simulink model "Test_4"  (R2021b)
settings: Solver=FixedStepAuto  StartTime=0.0  StopTime=1200
undefined symbols (not defined in the file): Ion, Lithium, Pe
libraries: fl_lib x31, nesl_utility x24, sdl_lib x11, simulink x5, simulink_extras x2, spsBatteryLib x1, spsCurrentVoltageSimscapeInterfaceLib x1, slpidlib x1, spspowerguiLib x1
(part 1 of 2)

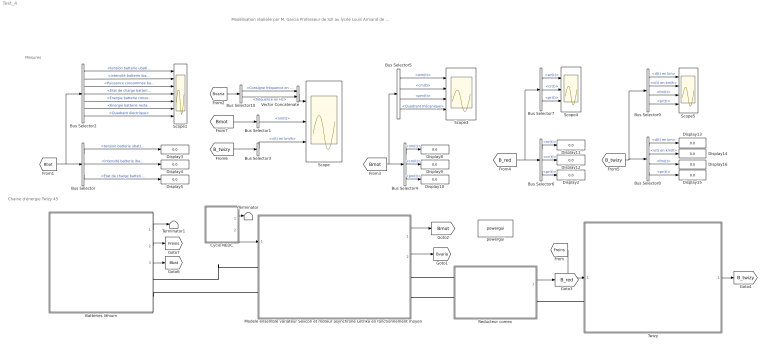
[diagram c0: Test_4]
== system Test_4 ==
  note: Mesures
  note: Chaine d'énergie Twizy 45
  note: Modélisation réalisée par M. Garcia Professeur de S2I au lycée Louis Armand de Nogent sur Marne
  Batteries lithium : Subsystem  mask{Ubat_n=54, Qbat_n=105, Soc_init=100, Soc_min=3}
      mask prompts: Ubat_n "Tension nominale batterie en V"; Qbat_n "Capacité nominale en A.h"; Soc_init "Etat de charge initial"; Soc_min "Seuil minimum en %"
  Bus Selector : BusSelector  OutputSignals=tension batterie ubat(t),intensité batterie ibat(t),Etat de charge batterie soc(t) en %
  Bus Selector1 : BusSelector  OutputSignals=nm(t)
  Bus Selector10 : BusSelector  OutputSignals=Consigne fréquence en Hz,fréquence en Hz
  Bus Selector2 : BusSelector  OutputSignals=tension batterie ubat(t),intensité batterie ibat(t),Puissance consommée batterie pbat(t) en W,Etat de charge batterie soc(t) en %,Energie batterie consommée wbat_cons(t) en Wh,Energie batterie restante wbat_rest(t) en Wh,Quadrant électrique
  Bus Selector3 : BusSelector  OutputSignals=v(t) en km/h
  Bus Selector4 : BusSelector  OutputSignals=nm(t),cm(t),pm(t)
  Bus Selector5 : BusSelector  OutputSignals=wm(t),cm(t),pm(t),Quadrant mécanique
  Bus Selector6 : BusSelector  OutputSignals=nr(t),cr(t),pr(t)
  Bus Selector7 : BusSelector  OutputSignals=wr(t),cr(t),pr(t)
  Bus Selector8 : BusSelector  OutputSignals=d(t) en km,v(t) en km/h,fm(t),pr(t)
  Bus Selector9 : BusSelector  OutputSignals=d(t) en km,v(t) en km/h,fm(t),pr(t)
  Cycle NEDC : Stateflow chart  TreatAsAtomicUnit=on
  Display{2..5,8..16} (13 alike) : Display
  Modele ensemble variateur Sevcon et moteur asynchrone Letrika en fonctionnement moyen : Subsystem  mask{Vbn=52, Tn=33, Nn=2050, fn=68.33, In=120, rend_mot=85, Jm=0.006, f_max_av=190, f_max_ar=54.8, rend_var=92, kp_n=1, ki_n=0.01, pas=0.5}
      mask prompts: Vbn "Tension bobinage nominale moteur en V"; Tn "Couple nominal en N.m"; Nn "Vitesse nominale moteur en tr/min"; fn "fréquence nominale moteur en Hz"; In "Intensité nominale moteur en A"; rend_mot "Rendement moteur en %"; Jm "Moment d'inertie moteur en kg.m²"; f_max_av "Fréquence maximale autorisée en marche avant en hz"; f_max_ar "Fréquence maximale autorisée en marche arrière en hz"; rend_var "Rendement variateur en %"; kp_n "Gain correcteur proportionnel"; ki_n "Gain correcteur intégral"; pas "Réglage pas solveur simscape"
  Reducteur comex : Subsystem  mask{ratio=(68*57)/(17*17), rend_red=96}
      mask prompts: ratio "Rapport de réduction"; rend_red "Rendement moyen transmission en %"
  Scope : Scope  NumInputPorts=3
  Scope1 : Scope  NumInputPorts=7
  Scope3 : Scope  NumInputPorts=4
  Scope4 : Scope  NumInputPorts=3
  Scope5 : Scope  NumInputPorts=4
  Terminator : Terminator
  Terminator1 : Terminator
  Twizy : Subsystem  mask{Vent_de_face=0, Pente=0, n=2, a=746, b=942, h=900, S=1.33, Cx=0.64, M_twizy=375, M_cond=80, M_pass=0, M_Batt=71, t_jantes_av=13, l_pneu_av=125, h_broul_av=80, Prav=2.5, t_jantes_ar=13, l_pneu_ar=145, h_broul_ar=80, Prar=2.5}
      mask prompts: Vent_de_face "Vent de face en km/h"; Pente "Pente de la route en %"; n "Nombre de roue par axe"; a "Distance estimée entre centre de gravitée et l'axe de la roue avant en mm"; b "Distance estimée entre centre de gravité e  et l'axe de la roue arrière en mm"; h "Hauteur estimée du centre de gravité en mm"; S "Surface frontale en m²"; Cx "Coefficient de trainée"; M_twizy "Masse twizy à vide en kg"; M_cond "Masse conducteur en kg"; M_pass "Masse passagers en kg"; M_Batt "Masse batteries en kg"; t_jantes_av "Taille jante en pouces"; l_pneu_av "Largeur en mm"; h_broul_av "Hauteur bande de roulement en %"; Prav "Pression pneus avant en bar"; t_jantes_ar "Taille jante en pouces"; l_pneu_ar "Largeur en mm"; h_broul_ar "Hauteur bande de roulement en %"; Prar "Pression pneus arrière en bar"
  Vector Concatenate : Concatenate
  powergui : spspowerguiLib/powergui  Priority=1  SimulationMode=Discrete  SampleTime=1  frequency=60  Iterations=50  frequencyindice=0  Pbase=100e6  ErrMax=1e-4  UnitsV=kV  UnitsW=MW  buscounter=0  FunctionMessages=off  echomessages=off  EnableUseOfTLC=off  CurrentSourceSwitches=off  DisableSnubberDevices=off  DisableRonSwitches=off  DisableVfSwitches=off  DisplayEquations=off  AutomaticDiscreteSolvers=off  SolverType=Tustin/Backward Euler (TBE)  Interpol=off  ExternalGateDelay=off  methode=off  Ts=100  x0status=blocks  SPID=on  SwTol=0  HookPort=off  NonlinearTolerance=1e-4  nMaxIteration=100  ContinueOnMaxIteration=off  RestoreLinks=warning  ResistiveCurrentMeasurement=off  Frange=[0:2:500]  Ylog=off  Xlog=on  ShowGrid=off  save=off  variable=ZData  structure=0  ZoomFFT=off  StartTime=0.0  cycles=1  DisplayStyle=1  fundamental=60  FreqAxis=off  MaxFrequency=1000  frequencyindicesteady=1  RmsSteady=1  display=off
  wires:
  Reducteur comex/1(Bus) -> [B_red]
  Twizy/1(Bus) -> [B_twizy]
  Modele ensemble variateur Sevcon et moteur asynchrone Letrika en fonctionnement moyen/1(Bus) -> [Bmot]
  Bus Selector/2 -> Display4/1  "<intensité batterie ibat(t)>"
  [Bbat] -> Bus Selector2/1, Bus Selector/1
  Bus Selector9/2 -> Scope5/2  "<v(t) en km/h>"
  Bus Selector9/4 -> Scope5/4  "<pr(t)>"
  Bus Selector8/2 -> Display14/1  "<v(t) en km/h>"
  Bus Selector6/2 -> Display12/1  "<cr(t)>"
  Bus Selector8/3 -> Display16/1  "<fm(t)>"
  Bus Selector7/1 -> Scope4/1  "<wr(t)>"
  Bus Selector8/1 -> Display13/1  "<d(t) en km>"
  Bus Selector4/3 -> Display10/1  "<pm(t)>"
  Bus Selector6/1 -> Display11/1  "<nr(t)>"
  Bus Selector5/3 -> Scope3/3  "<pm(t)>"
  Bus Selector5/2 -> Scope3/2  "<cm(t)>"
  Bus Selector6/3 -> Display2/1  "<pr(t)>"
  Bus Selector5/1 -> Scope3/1  "<wm(t)>"
  Bus Selector4/1 -> Display8/1  "<nm(t)>"
  [B_twizy] -> Bus Selector9/1, Bus Selector8/1
  Bus Selector2/1 -> Scope1/1  "<tension batterie ubat(t)>"
  [Bmot] -> Bus Selector4/1, Bus Selector5/1
  Bus Selector9/1 -> Scope5/1  "<d(t) en km>"
  [B_red] -> Bus Selector7/1, Bus Selector6/1
  Bus Selector7/3 -> Scope4/3  "<pr(t)>"
  Bus Selector2/2 -> Scope1/2  "<intensité batterie ibat(t)>"
  Bus Selector9/3 -> Scope5/3  "<fm(t)>"
  Bus Selector8/4 -> Display15/1  "<pr(t)>"
  Bus Selector2/3 -> Scope1/3  "<Puissance consommée batterie pbat(t) en W>"
  Bus Selector7/2 -> Scope4/2  "<cr(t)>"
  Bus Selector/1 -> Display3/1  "<tension batterie ubat(t)>"
  Bus Selector4/2 -> Display9/1  "<cm(t)>"
  Bus Selector/3 -> Display5/1  "<Etat de charge batterie soc(t) en %>"
  [Freins] -> Twizy/1(Forces freinages avant et arrières)
  Bus Selector2/4 -> Scope1/4  "<Etat de charge batterie soc(t) en %>"
  Modele ensemble variateur Sevcon et moteur asynchrone Letrika en fonctionnement moyen/2(Bus1) -> [Bvaria]
  [Bvaria] -> Bus Selector10/1
  [Bmot] -> Bus Selector1/1
  Bus Selector1/1 -> Scope/2  "<nm(t)>"
  [B_twizy] -> Bus Selector3/1
  Bus Selector3/1 -> Scope/3  "<v(t) en km/h>"
  Vector Concatenate/1 -> Scope/1
  Bus Selector10/1 -> Vector Concatenate/1  "<Consigne fréquence en Hz>"
  Bus Selector10/2 -> Vector Concatenate/2  "<fréquence en Hz>"
  Bus Selector2/7 -> Scope1/7  "<Quadrant électrique>"
  Bus Selector2/5 -> Scope1/5  "<Energie batterie consommée wbat_cons(t) en Wh>"
  Bus Selector2/6 -> Scope1/6  "<Energie batterie restante wbat_rest(t) en Wh>"
  Bus Selector5/4 -> Scope3/4  "<Quadrant mécanique>"
  Cycle NEDC/2(Consigne_acc) -> Modele ensemble variateur Sevcon et moteur asynchrone Letrika en fonctionnement moyen/1(Consigne Accélérateur en %)
  Cycle NEDC/1(Consigne) -> Terminator/1
  Batteries lithium/1(Stop) -> Terminator1/1
  Batteries lithium/3(Bus batterie) -> [Bbat]
  Batteries lithium/2(Freinage) -> [Freins]
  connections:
  Twizy/LConn1 -- Reducteur comex/RConn1
  Reducteur comex/LConn2 -- Modele ensemble variateur Sevcon et moteur asynchrone Letrika en fonctionnement moyen/RConn2
  Reducteur comex/LConn1 -- Modele ensemble variateur Sevcon et moteur asynchrone Letrika en fonctionnement moyen/RConn1
  Batteries lithium/RConn2 -- Modele ensemble variateur Sevcon et moteur asynchrone Letrika en fonctionnement moyen/LConn2
  Batteries lithium/RConn1 -- Modele ensemble variateur Sevcon et moteur asynchrone Letrika en fonctionnement moyen/LConn1

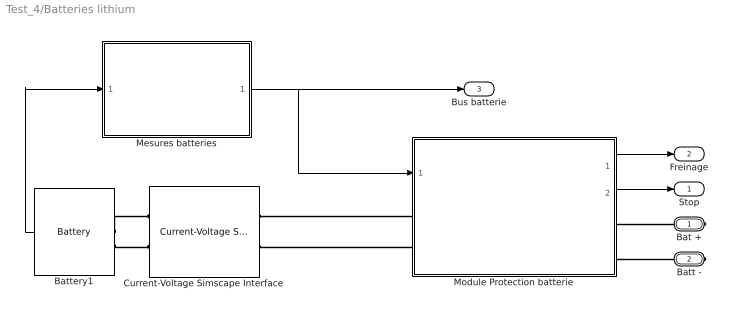
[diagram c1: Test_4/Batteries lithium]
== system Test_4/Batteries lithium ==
  Battery1 : spsBatteryLib/Battery  BatType=Lithium-Ion  ShowTempParam=off  ThermalPreset=no  ShowAgeParam=off  NomV=Ubat_n  NomQ=Qbat_n  SOC=Soc_init  Batt_Tr=30  PresetModel=on  MaxQ=105  MinV=40.5  FullV=62.8553  Dis_rate=45.6522  R=0.0051429  Normal_OP=94.9565  expZone="[58.3408       5.1587]"  current=[100 150 200]  Units=Time  Tci=20  NomT=20  T2=-30  MaxQ2=4.8  FullV2=7.1  Normal_OP2=5.655  expZone2="[6.58           1]"  Rca=0.6  ti=2000  Dp=0  Neq0=0  Tsim=1e6  Ta1=25  Qeol=5.4*0.9  Reol=0.013333*1.2  Char_age=[2.3478, 3]  Dis_age=[2.3478, 10]  N1=1500  N2=10500  N3=1000  N4=1400  Ta2=45  N5=950
  Current-Voltage Simscape Interface : spsCurrentVoltageSimscapeInterfaceLib/Current-Voltage Simscape Interface  DFT=off  FMode=Unit delay (discrete)  T=1e-6  Ts=-1  i0=0  v0=52  Sd=Simscape side  Measurements=off
  Mesures batteries : Subsystem
  Module Protection batterie : Subsystem
  Bat + : PMIOPort  Side=Right
  Batt - : PMIOPort  Port=2  Side=Right
  Stop : Outport  VectorParamsAs1DForOutWhenUnconnected=off
  Freinage : Outport  Port=2  VectorParamsAs1DForOutWhenUnconnected=off
  Bus batterie : Outport  Port=3  VectorParamsAs1DForOutWhenUnconnected=off
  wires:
  Battery1/1 -> Mesures batteries/1(Bus batteries)
  Mesures batteries/1(Bus_ batteries) -> Module Protection batterie/1(Bus batterie), Bus batterie/1
  Module Protection batterie/1(Freinage) -> Freinage/1
  Module Protection batterie/2(Stop) -> Stop/1
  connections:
  Battery1/LConn2 -- Current-Voltage Simscape Interface/LConn2
  Battery1/LConn1 -- Current-Voltage Simscape Interface/LConn1
  Module Protection batterie/RConn2 -- Batt -/RConn1
  Module Protection batterie/RConn1 -- Bat +/RConn1
  Module Protection batterie/LConn1 -- Current-Voltage Simscape Interface/RConn1
  Module Protection batterie/LConn2 -- Current-Voltage Simscape Interface/RConn2

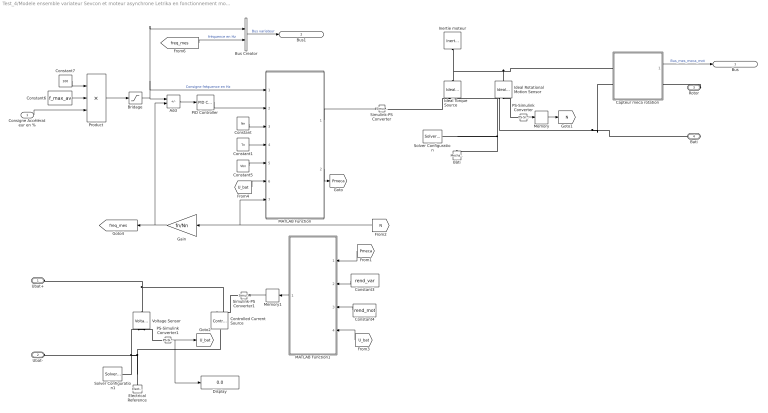
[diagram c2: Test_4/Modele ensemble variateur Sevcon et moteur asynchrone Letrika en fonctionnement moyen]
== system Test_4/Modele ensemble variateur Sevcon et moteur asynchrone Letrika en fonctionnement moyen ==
  Consigne Accélérateur en % : Inport
  Add : Sum  Inputs=+-
  Bridage : Saturate  UpperLimit=f_max_av  LowerLimit=-f_max_ar
  Bus Creator : BusCreator  Inputs=2
  Bâti : fl_lib/Mechanical/Rotational Elements/Mechanical Rotational Reference
  Capteur meca rotation : Subsystem
  Constant : Constant  Value=Nn
  Constant1 : Constant  Value=Tn
  Constant3 : Constant  Value=rend_var
  Constant4 : Constant  Value=rend_mot
  Constant5 : Constant  Value=Vbn
  Constant6 : Constant  Value=f_max_av
  Constant7 : Constant  Value=100
  Controlled Current Source : fl_lib/Electrical/Electrical Sources/Controlled Current Source
  Display : Display
  Electrical Reference : fl_lib/Electrical/Electrical Elements/Electrical Reference
  Gain : Gain  Gain=fn/Nn
  Ideal Rotational Motion Sensor : fl_lib/Mechanical/Mechanical Sensors/Ideal Rotational Motion Sensor  wrap_angle=simscape.enum.onoff.off  offset=0 rad
  Ideal Torque Source : fl_lib/Mechanical/Mechanical Sources/Ideal Torque Source
  Inertie moteur : fl_lib/Mechanical/Rotational Elements/Inertia  inertia=Jm kg*m^2  num_ports=foundation.enum.numPorts2.one  w_specify=off  w_priority=High  w=0 rad/s  w_nominal_specify=off  w_nominal_unit=rad/s  w_nominal_value=1  t_specify=off  t_priority=None  t=0 N*m  t_nominal_specify=off  t_nominal_unit=N*m  t_nominal_value=1
  MATLAB Function : MATLAB Function  TreatAsAtomicUnit=on
  MATLAB Function1 : MATLAB Function  TreatAsAtomicUnit=on
  Memory : Memory
  Memory1 : Memory
  PID Controller : slpidlib/PID Controller  Controller=PID  Form=Parallel  TimeDomain=Continuous-time  UseExternalTs=off  SampleTime=-1  IntegratorMethod=Forward Euler  FilterMethod=Forward Euler  ControllerParametersSource=internal  P=kp_n  I=ki_n  D=0  UseFilter=on  N=100  TunerSelectOption=Transfer Function Based (PID Tuner App)  InitialConditionSource=internal  InitialConditionForIntegrator=0  InitialConditionForFilter=0  DifferentiatorICPrevScaledInput=0  ExternalReset=none  TrackingMode=off  Kt=1  LimitOutput=off  SatLimitsSource=internal  UpperSaturationLimit=inf  LowerSaturationLimit=-inf  LinearizeAsGain=on  AntiWindupMode=none  Kb=1  POutMin=[]  POutMax=[]  IOutMin=[]  IOutMax=[]  DOutMin=[]  DOutMax=[]  NOutMin=[]  NOutMax=[]  SumOutMin=[]  SumOutMax=[]  SaturationOutMin=[]  SaturationOutMax=[]  PParamMin=[]  PParamMax=[]  IParamMin=[]  IParamMax=[]  DParamMin=[]  DParamMax=[]  NParamMin=[]  NParamMax=[]  KbParamMin=[]  KbParamMax=[]  KtParamMin=[]  KtParamMax=[]  KbOutMin=[]  KbOutMax=[]  KtOutMin=[]  KtOutMax=[]  IntegratorOutMin=[]  IntegratorOutMax=[]  FilterOutMin=[]  FilterOutMax=[]  SumI1OutMin=[]  SumI1OutMax=[]  SumI2OutMin=[]  SumI2OutMax=[]  SumI3OutMin=[]  SumI3OutMax=[]  SumI4OutMin=[]  SumI4OutMax=[]  SumDOutMin=[]  SumDOutMax=[]  DifferentiatorOutMin=[]  DifferentiatorOutMax=[]  FilterDiffOutCoefMin=[]  FilterDiffOutCoefMax=[]  ReciprocalOutMin=[]  ReciprocalOutMax=[]  SumDenOutMin=[]  SumDenOutMax=[]  SumNumOutMin=[]  SumNumOutMax=[]  DivideOutMin=[]  DivideOutMax=[]  UdiffTsProdOutMin=[]  UdiffTsProdOutMax=[]  NTsProdOutMin=[]  NTsProdOutMax=[]  UintegralTsProdOutMin=[]  UintegralTsProdOutMax=[]  UngainTsProdOutMin=[]  UngainTsProdOutMax=[]  IntegratorContinuousStateAttributes=''  IntegratorStateMustResolveToSignalObject=off  IntegratorRTWStateStorageClass=Auto  FilterContinuousStateAttributes=''  FilterStateMustResolveToSignalObject=off  FilterRTWStateStorageClass=Auto  ParallelPVariant=InternalParameters  IdealPVariant=Disabled  IVariant=InternalParameters  DVariant=InternalParameters  IntegratorVariant=Continuous  SatVariant=Disabled  AWVariant=Passthrough  PCopyVariant=Disabled  TRVariant=Disabled  FdbkBlocksVariant=Forward  IdealPFdbkVariant=Disabled  SatFdbkVariant=Disabled  DerivativeFilterVariant=ContFilter  NVariant=InternalParameters  NCopyVariant=Disabled  FilterICVariant=InternalICsFilter  IntegratorICVariant=InternalICs  ExternalResetVariant=Disabled  TRSumVariant=Passthrough  SumFdbkVariant=Disabled  SumVariant=Sum_PID  TsampFilterVariant=InternalTs  TsampNgainVariant=Passthrough  TsampIntegralVariant=Passthrough  ExternalSaturationOutDataTypeStr=Inherit: Same as second input
  PS-Simulink Converter : nesl_utility/PS-Simulink Converter  PhysicalDomain=network_engine_domain  SubClassName=ps_output  LeftPortType=input  RightPortType=output  PseudoPeriodic=off  Frequencies=[]  Unit=rpm  AffineConversion=off
  PS-Simulink Converter1 : nesl_utility/PS-Simulink Converter  PhysicalDomain=network_engine_domain  SubClassName=ps_output  LeftPortType=input  RightPortType=output  PseudoPeriodic=off  Frequencies=[]  Unit=V  AffineConversion=off
  Product : Product  Inputs=/**
  Simulink-PS Converter : nesl_utility/Simulink-PS Converter  PhysicalDomain=network_engine_domain  SubClassName=ps_input  LeftPortType=input  RightPortType=output  PseudoPeriodic=off  Frequencies=[]  NoiseDistribution=none  NoiseParameters=[]  Unit=N*m  AffineConversion=off  FilteringAndDerivatives=provide  SimscapeFilterOrder=1  InputFilterTimeConstant=0.001  UdotUserProvided=0
  Simulink-PS Converter1 : nesl_utility/Simulink-PS Converter  PhysicalDomain=network_engine_domain  SubClassName=ps_input  LeftPortType=input  RightPortType=output  PseudoPeriodic=off  Frequencies=[]  NoiseDistribution=none  NoiseParameters=[]  Unit=A  AffineConversion=off  FilteringAndDerivatives=provide  SimscapeFilterOrder=1  InputFilterTimeConstant=0.001  UdotUserProvided=0
  Solver Configuration : nesl_utility/Solver Configuration  PhysicalDomain=network_engine_domain  SubClassName=solver  LeftPortType=input  RightPortType=generic  Tones=[]  Harmonics=[]  SimulateNoise=off  Profile=off  UseLocalSampling=off  EnableSwitchedLinearOptims=on  FrequencyDomain=off  UseCCode=off  RelTol=0.001  AbsTol=1e-06  MinStep=1e-09  ToWorkspace=off  RevertToSquareIcSolve=off  NumHomotopyIterations=100  PhasorMode=off  PhasorModeNumHarmonics=1  DoDC=off  ResidualTolerance=1e-9  UseLocalSolver=on  LocalSolverChoice=NE_BACKWARD_EULER_ADVANCER  LocalSolverSampleTime=pas  DoFixedCost=on  MaxNonlinIter=3  MaxModeIter=2  ComputeImpulses=off  ImpulseIterations=2  LinearAlgebra=auto  EquationFormulation=NE_TIME_EF  DelaysMemoryBudget=1024  AutomaticFiltering=on  FilteringTimeConstant=0.001  PartitionStorageMethod=AS_NEEDED  PartitionMemoryBudget=1024  PartitionMethod=FAST
  Solver Configuration1 : nesl_utility/Solver Configuration  PhysicalDomain=network_engine_domain  SubClassName=solver  LeftPortType=input  RightPortType=generic  Tones=[]  Harmonics=[]  SimulateNoise=off  Profile=off  UseLocalSampling=off  EnableSwitchedLinearOptims=on  FrequencyDomain=off  UseCCode=off  RelTol=0.001  AbsTol=1e-06  MinStep=1e-09  ToWorkspace=off  RevertToSquareIcSolve=off  NumHomotopyIterations=100  PhasorMode=off  PhasorModeNumHarmonics=1  DoDC=off  ResidualTolerance=1e-9  UseLocalSolver=on  LocalSolverChoice=NE_BACKWARD_EULER_ADVANCER  LocalSolverSampleTime=pas  DoFixedCost=on  MaxNonlinIter=3  MaxModeIter=2  ComputeImpulses=off  ImpulseIterations=2  LinearAlgebra=auto  EquationFormulation=NE_TIME_EF  DelaysMemoryBudget=1024  AutomaticFiltering=on  FilteringTimeConstant=0.001  PartitionStorageMethod=AS_NEEDED  PartitionMemoryBudget=1024  PartitionMethod=FAST
  Voltage Sensor : fl_lib/Electrical/Electrical Sensors/Voltage Sensor
  Ubat+ : PMIOPort  Side=Left
  Ubat- : PMIOPort  Port=2  Side=Left
  Rotor : PMIOPort  Port=3  Side=Right
  Bati : PMIOPort  Port=4  Side=Right
  Bus : Outport  VectorParamsAs1DForOutWhenUnconnected=off
  Bus1 : Outport  Port=2  VectorParamsAs1DForOutWhenUnconnected=off
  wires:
  Capteur meca rotation/1(Out6) -> Bus/1  "Bus_mes_meca_mot"
  PS-Simulink Converter/1 -> Memory/1
  Constant/1 -> MATLAB Function/3(Nn)
  Constant1/1 -> MATLAB Function/4(Tn)
  [N] -> Gain/1, MATLAB Function/7(Nmes)
  Add/1 -> PID Controller/1
  PID Controller/1 -> MATLAB Function/2(T_in)
  Consigne Accélérateur en %/1 -> Product/3
  Memory/1 -> [N]
  MATLAB Function1/1(I_bat) -> Memory1/1
  MATLAB Function/2(P_meca) -> [Pmeca]
  [Pmeca] -> MATLAB Function1/1(Pmeca)
  Constant3/1 -> MATLAB Function1/2(rend_var)
  Constant4/1 -> MATLAB Function1/3(rend_mot)
  PS-Simulink Converter1/1 -> Display/1, [U_bat]
  [U_bat] -> MATLAB Function1/4(U_bat)
  [U_bat] -> MATLAB Function/6(U_bat)
  Constant5/1 -> MATLAB Function/5(Un)
  Gain/1 -> [freq_mes], Add/2
  Product/1 -> Bridage/1
  Constant6/1 -> Product/2
  Constant7/1 -> Product/1
  Bus Creator/1 -> Bus1/1  "Bus variateur"
  Bridage/1 -> Bus Creator/1, MATLAB Function/1(Consigne_frequence), Add/1  "Consigne fréquence en Hz"
  [freq_mes] -> Bus Creator/2  "fréquence en Hz"
  Memory1/1 -> Simulink-PS Converter1/1
  MATLAB Function/1(T_out) -> Simulink-PS Converter/1
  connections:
  Rotor/RConn1 -- Capteur meca rotation/RConn1
  Ideal Rotational Motion Sensor/RConn1 -- Bâti/LConn1 -- Solver Configuration/RConn1 -- Ideal Torque Source/RConn2 -- Bati/RConn1 -- Capteur meca rotation/LConn2
  Ideal Torque Source/LConn1 -- Inertie moteur/LConn1 -- Capteur meca rotation/LConn1 -- Ideal Rotational Motion Sensor/LConn1
  PS-Simulink Converter/LConn1 -- Ideal Rotational Motion Sensor/RConn2
  Simulink-PS Converter/RConn1 -- Ideal Torque Source/RConn1
  Ubat-/RConn1 -- Controlled Current Source/LConn1 -- Electrical Reference/LConn1 -- Solver Configuration1/RConn1 -- Voltage Sensor/RConn2
  PS-Simulink Converter1/LConn1 -- Voltage Sensor/RConn1
  Simulink-PS Converter1/RConn1 -- Controlled Current Source/RConn1
  Voltage Sensor/LConn1 -- Ubat+/RConn1 -- Controlled Current Source/RConn2

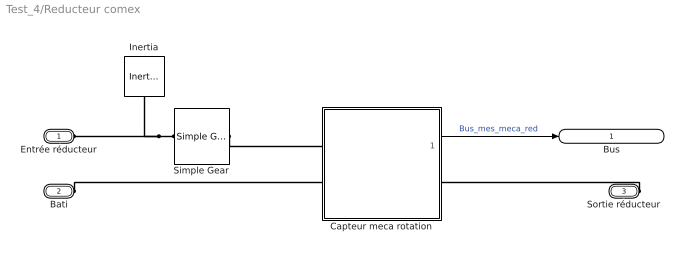
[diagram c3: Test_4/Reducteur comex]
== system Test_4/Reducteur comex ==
  Capteur meca rotation : Subsystem
  Inertia : fl_lib/Mechanical/Rotational Elements/Inertia  inertia=0.0085 kg*m^2  num_ports=foundation.enum.numPorts2.one  w_specify=off  w_priority=High  w=0 rad/s  w_nominal_specify=off  w_nominal_unit=rad/s  w_nominal_value=1  t_specify=off  t_priority=None  t=0 N*m  t_nominal_specify=off  t_nominal_unit=N*m  t_nominal_value=1
  Simple Gear : sdl_lib/Gears/Simple Gear  ratio=ratio  rotation_direction=3-2*(1)  friction_model=2  T_noload=0.1 N*m  T_nom=5 N*m  efficiency_nom=0.8  efficiency=rend_red/100  temperature_TLU=[280, 300, 320] K  load_TLU=[1, 5, 10] N*m  efficiency_TLU=[.95, .9, .85]  efficiency_TLU2=[.85, .8, .75; .95, .9, .85; .85, .8, .7]  w_thr=0.01 rad/s  pwr_thr=0.001 W  backlash_model=sdl.enum.backlashModel.Off  backlash_distance=1e-3 mm  x0=0 mm  r_base=0.1 m  hardstop_model=simscape.enum.hardstop.smooth  transition=1e-4 mm  backlash_stiffness=1e7 N/m  backlash_damping=1e6 N*s/m  e=0  v_tol=0.001 m/s  mu_visc=[0, 0] N*m/(rad/s)  enable_faults=0  efficiency_fault=0.05  external_fault=simscape.enum.onoff.off  temporal_fault=0  fault_time=5 s  fault_angles=pi / 12 rad  report_fault=(1)-1  thermal_mass=50 J/K  temperature_specify=off  temperature_priority=High  temperature=300 K  temperature_nominal_specify=off  temperature_nominal_unit=K  temperature_nominal_value=1  x_backlash_specify=off  x_backlash_priority=None  x_backlash=0 mm  x_backlash_nominal_specify=off  x_backlash_nominal_unit=mm  x_backlash_nominal_value=1  f_hardstop_specify=off  f_hardstop_priority=None  f_hardstop=0 N  f_hardstop_nominal_specify=off  f_hardstop_nominal_unit=N  f_hardstop_nominal_value=1  v_backlash_specify=off  v_backlash_priority=None  v_backlash=0 m/s  v_backlash_nominal_specify=off  v_backlash_nominal_unit=m/s  v_backlash_nominal_value=1
  Entrée réducteur : PMIOPort  Side=Left
  Bati : PMIOPort  Port=2  Side=Left
  Sortie réducteur : PMIOPort  Port=3  Side=Right
  Bus : Outport  VectorParamsAs1DForOutWhenUnconnected=off
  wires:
  Capteur meca rotation/1(Out6) -> Bus/1  "Bus_mes_meca_red"
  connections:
  Sortie réducteur/RConn1 -- Capteur meca rotation/RConn1
  Simple Gear/LConn1 -- Inertia/LConn1 -- Entrée réducteur/RConn1
  Bati/RConn1 -- Capteur meca rotation/LConn2
  Simple Gear/RConn1 -- Capteur meca rotation/LConn1

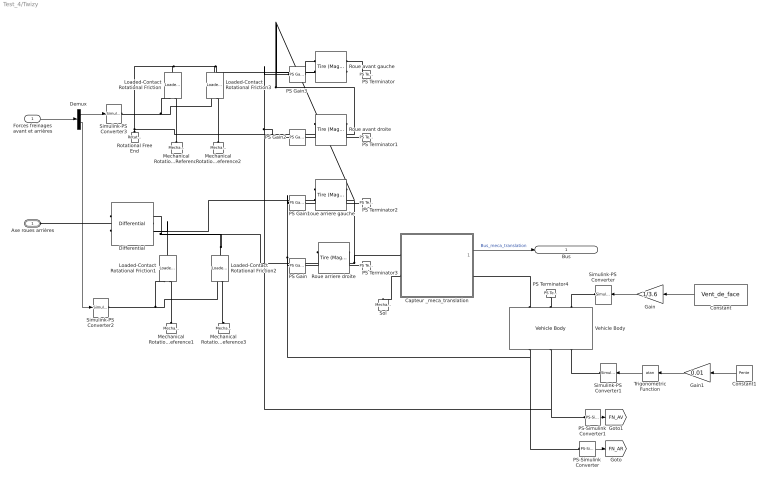
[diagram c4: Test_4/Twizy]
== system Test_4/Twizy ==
  Forces freinages avant et arrières : Inport
  Capteur _meca_translation : Subsystem
  Constant : Constant  Value=Vent_de_face
  Constant1 : Constant  Value=Pente
  Demux : Demux  Outputs=2
  Differential : sdl_lib/Gears/Differential  driveshaft_location=2  cd_ratio=1  friction_model=1  efficiency=[ 0.85 0.92 ]  temperature_TLU=[280, 300, 320] K  efficiency_ss_TLU=[.95, .9, .85]  efficiency_cd_TLU=[.95, .9, .85]  pwr_thr=[.001, .001] W  mu_visc=[ 0 0 ] N*m/(rad/s)  model_inertia=1  carrier_inertia=0.20 kg*m^2  planet_inertia=0.02 kg*m^2  thermal_mass=50 J/K  T_init=300 K
  Gain : Gain  Gain=1/3.6
  Gain1 : Gain  Gain=0.01
  Loaded-Contact Rotational Friction : sdl_lib/Brakes & Detents/Rotational/Loaded-Contact Rotational Friction  geometry_model=1  r_eff=280 mm  d_o=150 mm  d_i=100 mm  friction_model=1  mu_w_vector=[ 0 0.1 0.2 0.3 0.4 0.5 1 2 5 10 100 1000 ] rad/s  temperature_TLU=[280, 300, 320] K  mu_static=0.35  mu_static_vector=[.4, .38, .36]  mu_coulomb=0.3  mu_coulomb_vector=[ 0.29 0.28 0.26 0.22 0.21 0.2 0.2 0.19 0.19 0.19 0.19 0.19 ]  mu_coulomb_temp_vector=[.3, .28, .25]  mu_coulomb_matrix=[.34, .32, .3; .3, .28, .25; .25, .2, .15]  mu_interp_method=simscape.enum.interpolation.linear  mu_extrap_method=simscape.enum.extrapolation.linear  w_tol=0.001 rad/s  force_min=1 N  mu_visc=0 N*m/(rad/s)  initial_state_locked=0  enable_faults=simscape.enum.onoff.off  fault_type=sdl.enum.clutchFault.lock  external_fault=simscape.enum.onoff.off  temporal_fault=simscape.enum.onoff.off  fault_time=5 s  report_fault=simscape.enum.assert.action.none  thermal_mass=50 kJ/K  T_init=300 K
  Loaded-Contact Rotational Friction1 : sdl_lib/Brakes & Detents/Rotational/Loaded-Contact Rotational Friction  geometry_model=1  r_eff=280 mm  d_o=150 mm  d_i=100 mm  friction_model=1  mu_w_vector=[ 0 0.1 0.2 0.3 0.4 0.5 1 2 5 10 100 1000 ] rad/s  temperature_TLU=[280, 300, 320] K  mu_static=0.35  mu_static_vector=[.4, .38, .36]  mu_coulomb=0.3  mu_coulomb_vector=[ 0.29 0.28 0.26 0.22 0.21 0.2 0.2 0.19 0.19 0.19 0.19 0.19 ]  mu_coulomb_temp_vector=[.3, .28, .25]  mu_coulomb_matrix=[.34, .32, .3; .3, .28, .25; .25, .2, .15]  mu_interp_method=1  mu_extrap_method=1  w_tol=0.001 rad/s  force_min=1 N  mu_visc=0 N*m/(rad/s)  initial_state_locked=0  enable_faults=simscape.enum.onoff.off  fault_type=sdl.enum.clutchFault.lock  external_fault=simscape.enum.onoff.off  temporal_fault=simscape.enum.onoff.off  fault_time=5 s  report_fault=simscape.enum.assert.action.none  thermal_mass=50 kJ/K  T_init=300 K
  Loaded-Contact Rotational Friction2 : sdl_lib/Brakes & Detents/Rotational/Loaded-Contact Rotational Friction  geometry_model=1  r_eff=280 mm  d_o=150 mm  d_i=100 mm  friction_model=1  mu_w_vector=[ 0 0.1 0.2 0.3 0.4 0.5 1 2 5 10 100 1000 ] rad/s  temperature_TLU=[280, 300, 320] K  mu_static=0.35  mu_static_vector=[.4, .38, .36]  mu_coulomb=0.3  mu_coulomb_vector=[ 0.29 0.28 0.26 0.22 0.21 0.2 0.2 0.19 0.19 0.19 0.19 0.19 ]  mu_coulomb_temp_vector=[.3, .28, .25]  mu_coulomb_matrix=[.34, .32, .3; .3, .28, .25; .25, .2, .15]  mu_interp_method=1  mu_extrap_method=1  w_tol=0.001 rad/s  force_min=1 N  mu_visc=0 N*m/(rad/s)  initial_state_locked=0  enable_faults=simscape.enum.onoff.off  fault_type=sdl.enum.clutchFault.lock  external_fault=simscape.enum.onoff.off  temporal_fault=simscape.enum.onoff.off  fault_time=5 s  report_fault=simscape.enum.assert.action.none  thermal_mass=50 kJ/K  T_init=300 K
  Loaded-Contact Rotational Friction3 : sdl_lib/Brakes & Detents/Rotational/Loaded-Contact Rotational Friction  geometry_model=1  r_eff=280 mm  d_o=150 mm  d_i=100 mm  friction_model=1  mu_w_vector=[ 0 0.1 0.2 0.3 0.4 0.5 1 2 5 10 100 1000 ] rad/s  temperature_TLU=[280, 300, 320] K  mu_static=0.35  mu_static_vector=[.4, .38, .36]  mu_coulomb=0.3  mu_coulomb_vector=[ 0.29 0.28 0.26 0.22 0.21 0.2 0.2 0.19 0.19 0.19 0.19 0.19 ]  mu_coulomb_temp_vector=[.3, .28, .25]  mu_coulomb_matrix=[.34, .32, .3; .3, .28, .25; .25, .2, .15]  mu_interp_method=simscape.enum.interpolation.linear  mu_extrap_method=simscape.enum.extrapolation.linear  w_tol=0.001 rad/s  force_min=1 N  mu_visc=0 N*m/(rad/s)  initial_state_locked=0  enable_faults=simscape.enum.onoff.off  fault_type=sdl.enum.clutchFault.lock  external_fault=simscape.enum.onoff.off  temporal_fault=simscape.enum.onoff.off  fault_time=5 s  report_fault=simscape.enum.assert.action.none  thermal_mass=50 kJ/K  T_init=300 K
  Mechanical Rotational Reference{,1..3} (4 alike) : fl_lib/Mechanical/Rotational Elements/Mechanical Rotational Reference
  PS Gain{,1..3} (4 alike) : fl_lib/Physical Signals/Functions/PS Gain  gain=0.5
  PS Terminator{,1..4} (5 alike) : fl_lib/Physical Signals/Sinks/PS Terminator
  PS-Simulink Converter : nesl_utility/PS-Simulink Converter  PhysicalDomain=network_engine_domain  SubClassName=ps_output  LeftPortType=input  RightPortType=output  PseudoPeriodic=off  Frequencies=[]  Unit=N  AffineConversion=off
  PS-Simulink Converter1 : nesl_utility/PS-Simulink Converter  PhysicalDomain=network_engine_domain  SubClassName=ps_output  LeftPortType=input  RightPortType=output  PseudoPeriodic=off  Frequencies=[]  Unit=N  AffineConversion=off
  Rotational Free End : fl_lib/Mechanical/Rotational Elements/Rotational Free End  w_specify=off  w_priority=None  w=0 rad/s  w_nominal_specify=off  w_nominal_unit=rad/s  w_nominal_value=1
  Roue arriere droite : sdl_lib/Tires & Vehicles/Tire (Magic Formula)  parameterization=sdl.enum.magic_tire_model.constant  F_z1=3e+3 N  F_x1=3.5e+3 N  kappa1=10  B_m=10  C_m=1.9  D_m=1  E_m=0.97  fz0=4e+3 N  p_Cx=1.685  p_Dx=[ 1.21 -0.037 ]  p_Ex=[ 0.344 0.095 -0.02 0 ]  p_Kx=[ 21.51 -0.163 0.245 ]  p_Hx=[ -0.002 0.002 ]  p_Vx=[ 0 0 ]  r_e=(t_jantes_av*25.4+2*l_pneu_av*h_broul_av/100)/2 mm  model_compliance=sdl.enum.compliance.on  stiffness=1e+6 N/m  damping=1000 N/(m/s)  model_inertia=sdl.enum.model_inertia.on  inertia=0.12 kg*m^2  initial_velocity=0 rad/s  model_resistance=simscape.enum.onoff.on  resistance_model=sdl.enum.rollingResistanceParameterization.velocity  coeff=0.027*Pe  p_tire=Prar bar  alpha=-0.003  beta=0.97  coeff_a=84e-4*3.2  coeff_b=6.2e-4*3.2 s/m  coeff_c=1.6e-4 s^2/m^2  v_thr=1e-3 m/s  v_tr_thr=0.1 m/s
  Roue arriere gauche : sdl_lib/Tires & Vehicles/Tire (Magic Formula)  parameterization=sdl.enum.magic_tire_model.constant  F_z1=3e+3 N  F_x1=3.5e+3 N  kappa1=10  B_m=10  C_m=1.9  D_m=1  E_m=0.97  fz0=4e+3 N  p_Cx=1.685  p_Dx=[ 1.21 -0.037 ]  p_Ex=[ 0.344 0.095 -0.02 0 ]  p_Kx=[ 21.51 -0.163 0.245 ]  p_Hx=[ -0.002 0.002 ]  p_Vx=[ 0 0 ]  r_e=(t_jantes_av*25.4+2*l_pneu_av*h_broul_av/100)/2 mm  model_compliance=sdl.enum.compliance.on  stiffness=1e+6 N/m  damping=1000 N/(m/s)  model_inertia=sdl.enum.model_inertia.on  inertia=0.12 kg*m^2  initial_velocity=0 rad/s  model_resistance=simscape.enum.onoff.on  resistance_model=sdl.enum.rollingResistanceParameterization.velocity  coeff=0.027*Pe  p_tire=Prar bar  alpha=-0.003  beta=0.97  coeff_a=84e-4*3.2  coeff_b=6.2e-4*3.2 s/m  coeff_c=1.6e-4 s^2/m^2  v_thr=1e-3 m/s  v_tr_thr=0.1 m/s
  Roue avant droite : sdl_lib/Tires & Vehicles/Tire (Magic Formula)  parameterization=sdl.enum.magic_tire_model.constant  F_z1=3e+3 N  F_x1=3.5e+3 N  kappa1=10  B_m=10  C_m=1.9  D_m=1  E_m=0.97  fz0=4e+3 N  p_Cx=1.685  p_Dx=[ 1.21 -0.037 ]  p_Ex=[ 0.344 0.095 -0.02 0 ]  p_Kx=[ 21.51 -0.163 0.245 ]  p_Hx=[ -0.002 0.002 ]  p_Vx=[ 0 0 ]  r_e=(t_jantes_av*25.4+2*l_pneu_av*h_broul_av/100)/2 mm  model_compliance=sdl.enum.compliance.on  stiffness=1e+6 N/m  damping=1000 N/(m/s)  model_inertia=sdl.enum.model_inertia.on  inertia=0.12 kg*m^2  initial_velocity=0 rad/s  model_resistance=simscape.enum.onoff.on  resistance_model=sdl.enum.rollingResistanceParameterization.velocity  coeff=0.027*Pe  p_tire=Prav bar  alpha=-0.003  beta=0.97  coeff_a=84e-4*3.2  coeff_b=6.2e-4*3.2 s/m  coeff_c=1.6e-4 s^2/m^2  v_thr=1e-3 m/s  v_tr_thr=0.1 m/s
  Roue avant gauche : sdl_lib/Tires & Vehicles/Tire (Magic Formula)  parameterization=sdl.enum.magic_tire_model.constant  F_z1=3e+3 N  F_x1=3.5e+3 N  kappa1=10  B_m=10  C_m=1.9  D_m=1  E_m=0.97  fz0=4e+3 N  p_Cx=1.685  p_Dx=[ 1.21 -0.037 ]  p_Ex=[ 0.344 0.095 -0.02 0 ]  p_Kx=[ 21.51 -0.163 0.245 ]  p_Hx=[ -0.002 0.002 ]  p_Vx=[ 0 0 ]  r_e=(t_jantes_av*25.4+2*l_pneu_av*h_broul_av/100)/2 mm  model_compliance=sdl.enum.compliance.on  stiffness=1e+6 N/m  damping=1000 N/(m/s)  model_inertia=sdl.enum.model_inertia.on  inertia=0.12 kg*m^2  initial_velocity=0 rad/s  model_resistance=simscape.enum.onoff.on  resistance_model=sdl.enum.rollingResistanceParameterization.velocity  coeff=0.027*Pe  p_tire=Prav bar  alpha=-0.003  beta=0.97  coeff_a=84e-4*3.2  coeff_b=6.2e-4*3.2 s/m  coeff_c=1.6e-4 s^2/m^2  v_thr=1e-3 m/s  v_tr_thr=0.1 m/s
  Simulink-PS Converter : nesl_utility/Simulink-PS Converter  PhysicalDomain=network_engine_domain  SubClassName=ps_input  LeftPortType=input  RightPortType=output  PseudoPeriodic=off  Frequencies=[]  NoiseDistribution=none  NoiseParameters=[]  Unit=m/s  AffineConversion=off  FilteringAndDerivatives=zero  SimscapeFilterOrder=1  InputFilterTimeConstant=0.001  UdotUserProvided=1
  Simulink-PS Converter1 : nesl_utility/Simulink-PS Converter  PhysicalDomain=network_engine_domain  SubClassName=ps_input  LeftPortType=input  RightPortType=output  PseudoPeriodic=off  Frequencies=[]  NoiseDistribution=none  NoiseParameters=[]  Unit=rad  AffineConversion=off  FilteringAndDerivatives=zero  SimscapeFilterOrder=1  InputFilterTimeConstant=0.001  UdotUserProvided=1
  Simulink-PS Converter2 : nesl_utility/Simulink-PS Converter  PhysicalDomain=network_engine_domain  SubClassName=ps_input  LeftPortType=input  RightPortType=output  PseudoPeriodic=off  Frequencies=[]  NoiseDistribution=none  NoiseParameters=[]  Unit=N  AffineConversion=off  FilteringAndDerivatives=zero  SimscapeFilterOrder=1  InputFilterTimeConstant=0.001  UdotUserProvided=1
  Simulink-PS Converter3 : nesl_utility/Simulink-PS Converter  PhysicalDomain=network_engine_domain  SubClassName=ps_input  LeftPortType=input  RightPortType=output  PseudoPeriodic=off  Frequencies=[]  NoiseDistribution=none  NoiseParameters=[]  Unit=N  AffineConversion=off  FilteringAndDerivatives=zero  SimscapeFilterOrder=1  InputFilterTimeConstant=0.001  UdotUserProvided=1
  Sol : fl_lib/Mechanical/Translational Elements/Mechanical Translational Reference
  Trigonometric Function : Trigonometry  Operator=atan
  Vehicle Body : sdl_lib/Tires & Vehicles/Vehicle Body  mass=M_twizy+M_cond+M_pass+M_Batt kg  n_w=n  x_f=a mm  x_r=b mm  y_c=h mm  mass_var=simscape.enum.onoff.off  g=9.81 m/s^2  liftoff_warning=simscape.enum.onoff.off  area=S m^2  Cd=Cx  rho=1.18 kg/m^3  model_pitch=simscape.enum.onoff.on  inertia=4000 kg*m^2  suspension_model=sdl.enum.linearTLU.linear  k_f=1e4 N/m  b_f=1e4 N/(m/s)  k_r=1e4 N/m  b_r=1e4 N/(m/s)  k_f_TLU=[-2000, -1000, 0, 1000, 2000] N  x_f_TLU=[-.4, -.2, 0, .2, .4] m  b_f_TLU=[-200, -100, 0, 100, 200] N  v_f_TLU=[-4, -2, 0, 2, 4] m/s  k_r_TLU=[-2000, -1000, 0, 1000, 2000] N  x_r_TLU=[-.4, -.2, 0, .2, .4] m  b_r_TLU=[-200, -100, 0, 100, 200] N  v_r_TLU=[-4, -2, 0, 2, 4] m/s  interp_method=simscape.enum.interpolation.linear  extrap_method=simscape.enum.extrapolation.linear  model_hardstop=simscape.enum.onoff.off  upper_bound_f=.25 m  lower_bound_f=-.25 m  stop_k_f=1e6 N/m  stop_b_f=150 N/(m/s)  upper_bound_r=.25 m  lower_bound_r=-.25 m  stop_k_r=1e6 N/m  stop_b_r=150 N/(m/s)  initial_pitch=0 rad  initial_pitch_rate=0 rad/s  v_specify=on  v_priority=High  v=0 m/s  v_nominal_specify=off  v_nominal_unit=m/s  v_nominal_value=1
  Axe roues arrières : PMIOPort  Side=Left
  Bus : Outport  VectorParamsAs1DForOutWhenUnconnected=off
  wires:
  Capteur _meca_translation/1(Out6) -> Bus/1  "Bus_meca_translation"
  Constant/1 -> Gain/1
  Constant1/1 -> Gain1/1
  PS-Simulink Converter1/1 -> [FN_AV]
  PS-Simulink Converter/1 -> [FN_AR]
  Gain/1 -> Simulink-PS Converter/1
  Gain1/1 -> Trigonometric Function/1
  Trigonometric Function/1 -> Simulink-PS Converter1/1
  Demux/2 -> Simulink-PS Converter2/1
  Forces freinages avant et arrières/1 -> Demux/1
  Demux/1 -> Simulink-PS Converter3/1
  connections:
  Capteur _meca_translation/LConn2 -- Sol/LConn1
  Vehicle Body/LConn1 -- Capteur _meca_translation/RConn1
  Differential/RConn2 -- Loaded-Contact Rotational Friction1/RConn1 -- Roue arriere gauche/LConn2
  Vehicle Body/LConn3 -- Simulink-PS Converter/RConn1
  Vehicle Body/RConn3 -- Simulink-PS Converter1/RConn1
  PS Gain3/RConn1 -- Roue avant gauche/LConn1
  Vehicle Body/RConn1 -- PS-Simulink Converter/LConn1 -- PS Gain/LConn1 -- PS Gain1/LConn1
  Simulink-PS Converter2/RConn1 -- Loaded-Contact Rotational Friction1/LConn1 -- Loaded-Contact Rotational Friction2/LConn1
  Roue arriere gauche/RConn2 -- Roue avant droite/RConn2 -- Roue avant gauche/RConn2 -- Capteur _meca_translation/LConn1 -- Roue arriere droite/RConn2
  Rotational Free End/LConn1 -- Roue avant gauche/LConn2 -- Loaded-Contact Rotational Friction3/RConn1 -- Loaded-Contact Rotational Friction/RConn1 -- Roue avant droite/LConn2
  PS Terminator/LConn1 -- Roue avant gauche/RConn1
  Roue avant droite/RConn1 -- PS Terminator1/LConn1
  Roue arriere gauche/RConn1 -- PS Terminator2/LConn1
  Roue arriere droite/RConn1 -- PS Terminator3/LConn1
  Mechanical Rotational Reference/LConn1 -- Loaded-Contact Rotational Friction/LConn2
  Mechanical Rotational Reference1/LConn1 -- Loaded-Contact Rotational Friction1/LConn2
  PS Terminator4/LConn1 -- Vehicle Body/LConn2
  Simulink-PS Converter3/RConn1 -- Loaded-Contact Rotational Friction3/LConn1 -- Loaded-Contact Rotational Friction/LConn1
  Differential/LConn1 -- Axe roues arrières/RConn1
  Differential/RConn1 -- Loaded-Contact Rotational Friction2/RConn1 -- Roue arriere droite/LConn2
  Mechanical Rotational Reference2/LConn1 -- Loaded-Contact Rotational Friction3/LConn2
  Loaded-Contact Rotational Friction2/LConn2 -- Mechanical Rotational Reference3/LConn1
  Roue arriere droite/LConn1 -- PS Gain/RConn1
  Roue arriere gauche/LConn1 -- PS Gain1/RConn1
  Roue avant droite/LConn1 -- PS Gain2/RConn1
  Vehicle Body/RConn2 -- PS-Simulink Converter1/LConn1 -- PS Gain2/LConn1 -- PS Gain3/LConn1

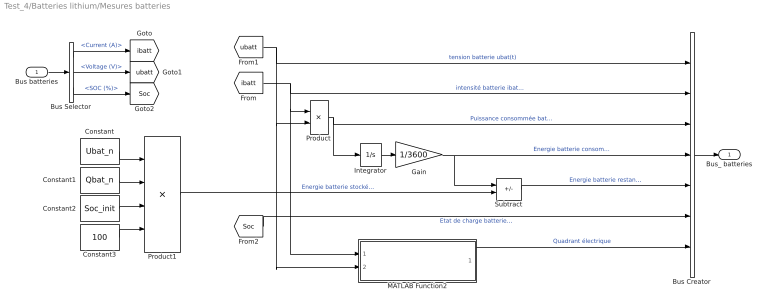
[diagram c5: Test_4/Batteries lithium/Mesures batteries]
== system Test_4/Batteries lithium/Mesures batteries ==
  Bus batteries : Inport
  Bus Creator : BusCreator  Inputs=7
  Bus Selector : BusSelector  OutputSignals=Current (A),Voltage (V),SOC (%)
  Constant : Constant  Value=Ubat_n
  Constant1 : Constant  Value=Qbat_n
  Constant2 : Constant  Value=Soc_init
  Constant3 : Constant  Value=100
  Gain : Gain  Gain=1/3600
  Integrator : Integrator
  MATLAB Function2 : MATLAB Function  TreatAsAtomicUnit=on
  Product : Product
  Product1 : Product  Inputs=***/
  Subtract : Sum  Inputs=-+
  Bus_ batteries : Outport  VectorParamsAs1DForOutWhenUnconnected=off
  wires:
  Bus batteries/1 -> Bus Selector/1
  Product/1 -> Bus Creator/3, Integrator/1  "Puissance consommée batterie pbat(t) en W"
  Bus Creator/1 -> Bus_ batteries/1
  Integrator/1 -> Gain/1
  Gain/1 -> Bus Creator/4, Subtract/1  "Energie batterie consommée wbat_cons(t) en Wh"
  [ibatt] -> MATLAB Function2/1(I_bat), Product/1, Bus Creator/2  "intensité batterie ibat(t)"
  Bus Selector/1 -> [ibatt]  "<Current (A)>"
  Bus Selector/2 -> [ubatt]  "<Voltage (V)>"
  [ubatt] -> MATLAB Function2/2(U_bat), Product/2, Bus Creator/1  "tension batterie ubat(t)"
  Bus Selector/3 -> [Soc]  "<SOC (%)>"
  [Soc] -> Bus Creator/6  "Etat de charge batterie soc(t) en %"
  MATLAB Function2/1(Quadrant_elec) -> Bus Creator/7  "Quadrant électrique"
  Constant/1 -> Product1/1
  Constant1/1 -> Product1/2
  Constant2/1 -> Product1/3
  Constant3/1 -> Product1/4
  Subtract/1 -> Bus Creator/5  "Energie batterie restante wbat_rest(t) en Wh"
  Product1/1 -> Subtract/2  "Energie batterie stockée wstock_batt(t) en Wh"

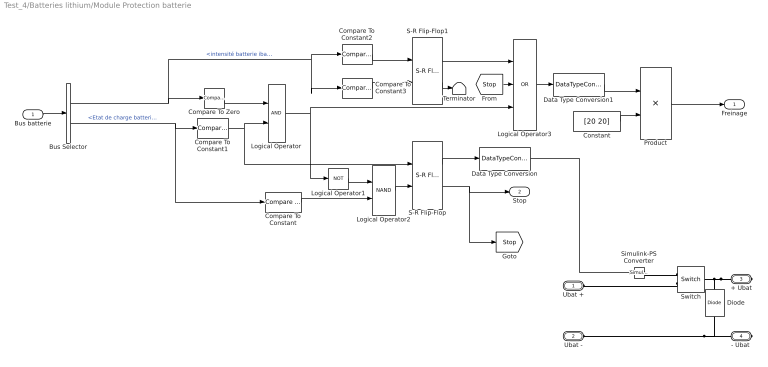
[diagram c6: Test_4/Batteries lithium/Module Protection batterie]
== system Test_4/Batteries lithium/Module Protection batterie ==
  Bus batterie : Inport
  Bus Selector : BusSelector  OutputSignals=intensité batterie ibat(t),Etat de charge batterie soc(t) en %
  Compare To Constant : simulink/Logic and Bit Operations/Compare To Constant  relop=>  const=Soc_min  OutDataTypeStr=boolean
  Compare To Constant1 : simulink/Logic and Bit Operations/Compare To Constant  relop=>=  const=100  OutDataTypeStr=boolean
  Compare To Constant2 : simulink/Logic and Bit Operations/Compare To Constant  relop=<=  const=-205  OutDataTypeStr=boolean
  Compare To Constant3 : simulink/Logic and Bit Operations/Compare To Constant  relop=>=  const=-185  OutDataTypeStr=boolean
  Compare To Zero : simulink/Logic and Bit Operations/Compare To Zero  relop=<  OutDataTypeStr=boolean
  Constant : Constant  Value=[20 20]
  Data Type Conversion : DataTypeConversion  OutDataTypeStr=double
  Data Type Conversion1 : DataTypeConversion  OutDataTypeStr=double
  Diode : fl_lib/Electrical/Electrical Elements/Diode  Vf=0.6 V  Ron=0.3 Ohm  Goff=1e-8 1/Ohm  i_specify=off  i_priority=None  i=0 A  i_nominal_specify=off  i_nominal_unit=A  i_nominal_value=1  v_specify=off  v_priority=None  v=0 V  v_nominal_specify=off  v_nominal_unit=V  v_nominal_value=1
  Logical Operator : Logic  AllPortsSameDT=off  OutDataTypeStr=boolean
  Logical Operator1 : Logic  Operator=NOT  AllPortsSameDT=off  OutDataTypeStr=boolean
  Logical Operator2 : Logic  Operator=NAND  AllPortsSameDT=off  OutDataTypeStr=boolean
  Logical Operator3 : Logic  Operator=OR  Inputs=3  AllPortsSameDT=off  OutDataTypeStr=boolean
  Product : Product
  S-R Flip-Flop : simulink_extras/Flip Flops/S-R Flip-Flop  initial_condition=1
  S-R Flip-Flop1 : simulink_extras/Flip Flops/S-R Flip-Flop  initial_condition=1
  Simulink-PS Converter : nesl_utility/Simulink-PS Converter  PhysicalDomain=network_engine_domain  SubClassName=ps_input  LeftPortType=input  RightPortType=output  PseudoPeriodic=off  Frequencies=[]  NoiseDistribution=none  NoiseParameters=[]  Unit=1  AffineConversion=off  FilteringAndDerivatives=provide  SimscapeFilterOrder=1  InputFilterTimeConstant=0.001  UdotUserProvided=0
  Switch : fl_lib/Electrical/Electrical Elements/Switch  R_closed=0.01 Ohm  G_open=1e-8 1/Ohm  Threshold=0.5  i_specify=off  i_priority=None  i=0 A  i_nominal_specify=off  i_nominal_unit=A  i_nominal_value=1  v_specify=off  v_priority=None  v=0 V  v_nominal_specify=off  v_nominal_unit=V  v_nominal_value=1
  Terminator : Terminator
  Ubat + : PMIOPort  Side=Left
  Ubat - : PMIOPort  Port=2  Side=Left
  + Ubat : PMIOPort  Port=3  Side=Right
  "- Ubat " : PMIOPort  Port=4  Side=Right
  Freinage : Outport  VectorParamsAs1DForOutWhenUnconnected=off
  Stop : Outport  Port=2  VectorParamsAs1DForOutWhenUnconnected=off
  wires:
  Bus Selector/2 -> Compare To Constant/1, Compare To Constant1/1  "<Etat de charge batterie soc(t) en %>"
  Compare To Constant/1 -> Logical Operator2/2
  Compare To Constant1/1 -> S-R Flip-Flop/1, Logical Operator/2
  Bus Selector/1 -> Compare To Constant3/1, Compare To Constant2/1, Compare To Zero/1  "<intensité batterie ibat(t)>"
  Compare To Zero/1 -> Logical Operator/1
  Logical Operator/1 -> Logical Operator1/1, Logical Operator3/3
  Data Type Conversion1/1 -> Product/1
  Logical Operator1/1 -> Logical Operator2/1
  Logical Operator2/1 -> S-R Flip-Flop/2
  Product/1 -> Freinage/1
  Constant/1 -> Product/2
  Bus batterie/1 -> Bus Selector/1
  Data Type Conversion/1 -> Simulink-PS Converter/1
  S-R Flip-Flop/2 -> [Stop], Stop/1
  S-R Flip-Flop/1 -> Data Type Conversion/1
  Logical Operator3/1 -> Data Type Conversion1/1
  [Stop] -> Logical Operator3/2
  Compare To Constant2/1 -> S-R Flip-Flop1/1
  S-R Flip-Flop1/1 -> Logical Operator3/1
  Compare To Constant3/1 -> S-R Flip-Flop1/2
  S-R Flip-Flop1/2 -> Terminator/1
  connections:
  + Ubat/RConn1 -- Switch/LConn1 -- Diode/RConn1
  Simulink-PS Converter/RConn1 -- Switch/RConn1
  Ubat -/RConn1 -- "- Ubat "/RConn1 -- Diode/LConn1
  Switch/RConn2 -- Ubat +/RConn1

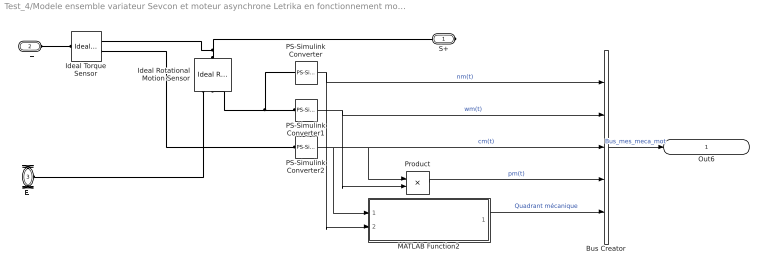
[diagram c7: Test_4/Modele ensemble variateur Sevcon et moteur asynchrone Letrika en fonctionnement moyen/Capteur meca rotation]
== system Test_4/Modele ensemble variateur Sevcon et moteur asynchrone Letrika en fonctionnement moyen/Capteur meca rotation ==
  Bus Creator : BusCreator  Inputs=5
  Ideal Rotational Motion Sensor : fl_lib/Mechanical/Mechanical Sensors/Ideal Rotational Motion Sensor  wrap_angle=simscape.enum.onoff.off  offset=0 rad
  Ideal Torque Sensor : fl_lib/Mechanical/Mechanical Sensors/Ideal Torque Sensor
  MATLAB Function2 : MATLAB Function  TreatAsAtomicUnit=on
  PS-Simulink Converter : nesl_utility/PS-Simulink Converter  PhysicalDomain=network_engine_domain  SubClassName=ps_output  LeftPortType=input  RightPortType=output  PseudoPeriodic=off  Frequencies=[]  Unit=rpm  AffineConversion=off
  PS-Simulink Converter1 : nesl_utility/PS-Simulink Converter  PhysicalDomain=network_engine_domain  SubClassName=ps_output  LeftPortType=input  RightPortType=output  PseudoPeriodic=off  Frequencies=[]  Unit=rad/s  AffineConversion=off
  PS-Simulink Converter2 : nesl_utility/PS-Simulink Converter  PhysicalDomain=network_engine_domain  SubClassName=ps_output  LeftPortType=input  RightPortType=output  PseudoPeriodic=off  Frequencies=[]  Unit=N*m  AffineConversion=off
  Product : Product
  S+ : PMIOPort  Side=Right
  E+ : PMIOPort  Port=2  Side=Left
  E- : PMIOPort  Port=3  Side=Left
  Out6 : Outport  VectorParamsAs1DForOutWhenUnconnected=off
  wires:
  PS-Simulink Converter/1 -> MATLAB Function2/2(Nm), Bus Creator/1  "nm(t)"
  Product/1 -> Bus Creator/4  "pm(t)"
  Bus Creator/1 -> Out6/1  "Bus_mes_meca_mot"
  PS-Simulink Converter1/1 -> Product/2, Bus Creator/2  "wm(t)"
  PS-Simulink Converter2/1 -> MATLAB Function2/1(Cm), Product/1, Bus Creator/3  "cm(t)"
  MATLAB Function2/1(Quadrant_meca) -> Bus Creator/5  "Quadrant mécanique"
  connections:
  PS-Simulink Converter2/LConn1 -- Ideal Torque Sensor/RConn2
  Ideal Rotational Motion Sensor/LConn1 -- S+/RConn1 -- Ideal Torque Sensor/RConn1
  PS-Simulink Converter1/LConn1 -- Ideal Rotational Motion Sensor/RConn2 -- PS-Simulink Converter/LConn1
  Ideal Torque Sensor/LConn1 -- E+/RConn1
  Ideal Rotational Motion Sensor/RConn1 -- E-/RConn1

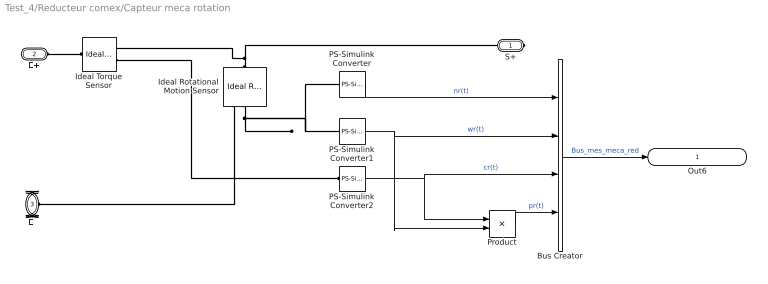
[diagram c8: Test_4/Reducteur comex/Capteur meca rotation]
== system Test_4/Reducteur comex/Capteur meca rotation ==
  Bus Creator : BusCreator  Inputs=4
  Ideal Rotational Motion Sensor : fl_lib/Mechanical/Mechanical Sensors/Ideal Rotational Motion Sensor  wrap_angle=simscape.enum.onoff.off  offset=0 rad
  Ideal Torque Sensor : fl_lib/Mechanical/Mechanical Sensors/Ideal Torque Sensor
  PS-Simulink Converter : nesl_utility/PS-Simulink Converter  PhysicalDomain=network_engine_domain  SubClassName=ps_output  LeftPortType=input  RightPortType=output  PseudoPeriodic=off  Frequencies=[]  Unit=rpm  AffineConversion=off
  PS-Simulink Converter1 : nesl_utility/PS-Simulink Converter  PhysicalDomain=network_engine_domain  SubClassName=ps_output  LeftPortType=input  RightPortType=output  PseudoPeriodic=off  Frequencies=[]  Unit=rad/s  AffineConversion=off
  PS-Simulink Converter2 : nesl_utility/PS-Simulink Converter  PhysicalDomain=network_engine_domain  SubClassName=ps_output  LeftPortType=input  RightPortType=output  PseudoPeriodic=off  Frequencies=[]  Unit=N*m  AffineConversion=off
  Product : Product
  S+ : PMIOPort  Side=Right
  E+ : PMIOPort  Port=2  Side=Left
  E- : PMIOPort  Port=3  Side=Left
  Out6 : Outport  VectorParamsAs1DForOutWhenUnconnected=off
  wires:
  PS-Simulink Converter/1 -> Bus Creator/1  "nr(t)"
  Product/1 -> Bus Creator/4  "pr(t)"
  Bus Creator/1 -> Out6/1  "Bus_mes_meca_red"
  PS-Simulink Converter1/1 -> Product/2, Bus Creator/2  "wr(t)"
  PS-Simulink Converter2/1 -> Product/1, Bus Creator/3  "cr(t)"
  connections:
  PS-Simulink Converter2/LConn1 -- Ideal Torque Sensor/RConn2
  Ideal Rotational Motion Sensor/LConn1 -- Ideal Torque Sensor/RConn1 -- S+/RConn1
  Ideal Rotational Motion Sensor/RConn2 -- PS-Simulink Converter1/LConn1 -- PS-Simulink Converter/LConn1
  Ideal Torque Sensor/LConn1 -- E+/RConn1
  Ideal Rotational Motion Sensor/RConn1 -- E-/RConn1

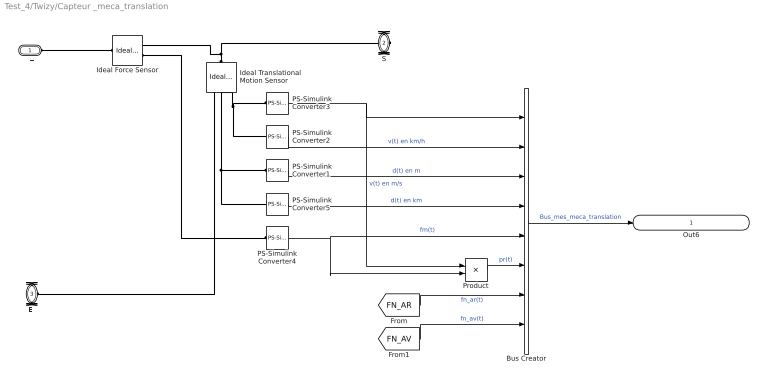
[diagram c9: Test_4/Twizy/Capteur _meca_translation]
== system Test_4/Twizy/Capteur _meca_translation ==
  Bus Creator : BusCreator  Inputs=8
  Ideal Force Sensor : fl_lib/Mechanical/Mechanical Sensors/Ideal Force Sensor
  Ideal Translational Motion Sensor : fl_lib/Mechanical/Mechanical Sensors/Ideal Translational Motion Sensor  offset=0 m
  PS-Simulink Converter1 : nesl_utility/PS-Simulink Converter  PhysicalDomain=network_engine_domain  SubClassName=ps_output  LeftPortType=input  RightPortType=output  PseudoPeriodic=off  Frequencies=[]  Unit=m  AffineConversion=off
  PS-Simulink Converter2 : nesl_utility/PS-Simulink Converter  PhysicalDomain=network_engine_domain  SubClassName=ps_output  LeftPortType=input  RightPortType=output  PseudoPeriodic=off  Frequencies=[]  Unit=km/hr  AffineConversion=off
  PS-Simulink Converter3 : nesl_utility/PS-Simulink Converter  PhysicalDomain=network_engine_domain  SubClassName=ps_output  LeftPortType=input  RightPortType=output  PseudoPeriodic=off  Frequencies=[]  Unit=m/s  AffineConversion=off
  PS-Simulink Converter4 : nesl_utility/PS-Simulink Converter  PhysicalDomain=network_engine_domain  SubClassName=ps_output  LeftPortType=input  RightPortType=output  PseudoPeriodic=off  Frequencies=[]  Unit=N  AffineConversion=off
  PS-Simulink Converter5 : nesl_utility/PS-Simulink Converter  PhysicalDomain=network_engine_domain  SubClassName=ps_output  LeftPortType=input  RightPortType=output  PseudoPeriodic=off  Frequencies=[]  Unit=km  AffineConversion=off
  Product : Product
  E+ : PMIOPort  Side=Left
  S : PMIOPort  Port=2  Side=Right
  E- : PMIOPort  Port=3  Side=Left
  Out6 : Outport  VectorParamsAs1DForOutWhenUnconnected=off
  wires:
  PS-Simulink Converter3/1 -> Product/1, Bus Creator/1  "v(t) en m/s"
  PS-Simulink Converter4/1 -> Bus Creator/5, Product/2  "fm(t)"
  Product/1 -> Bus Creator/6  "pr(t)"
  Bus Creator/1 -> Out6/1  "Bus_mes_meca_translation"
  PS-Simulink Converter1/1 -> Bus Creator/3  "d(t) en m"
  [FN_AR] -> Bus Creator/7  "fn_ar(t)"
  [FN_AV] -> Bus Creator/8  "fn_av(t)"
  PS-Simulink Converter2/1 -> Bus Creator/2  "v(t) en km/h"
  PS-Simulink Converter5/1 -> Bus Creator/4  "d(t) en km"
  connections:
  PS-Simulink Converter4/LConn1 -- Ideal Force Sensor/RConn2
  Ideal Translational Motion Sensor/LConn1 -- Ideal Force Sensor/RConn1 -- S/RConn1
  PS-Simulink Converter3/LConn1 -- PS-Simulink Converter2/LConn1 -- Ideal Translational Motion Sensor/RConn2
  Ideal Force Sensor/LConn1 -- E+/RConn1
  Ideal Translational Motion Sensor/RConn1 -- E-/RConn1
  PS-Simulink Converter1/LConn1 -- Ideal Translational Motion Sensor/RConn3 -- PS-Simulink Converter5/LConn1

== matlab function Test_4/Modele ensemble variateur Sevcon et moteur asynchrone Letrika
en fonctionnement moyen/MATLAB Function ==
function [T_out,P_meca]= fcn(Consigne_frequence, T_in,Nn,Tn,Un,U_bat,Nmes)
if U_bat <= Un
    k_corr = (U_bat/Un).^2;
else
    k_corr = 1;
end
P_max = Tn*(2*pi*Nn/60)*k_corr;

if Consigne_frequence~=0
    if abs(Nmes)<=Nn
        if abs(T_in)>=Tn*k_corr
            T_out=Tn*sign(T_in)*k_corr;
        else
            T_out=T_in*k_corr;
        end
    else
        if abs(T_in)>=P_max/(2*pi*Nmes/60)
            T_out=sign(T_in)*P_max/(2*pi*Nmes/60);
        else
            T_out=T_in;
        end
    end
else
    T_out=0;
end

P_meca = T_out*2*pi*Nmes/60;

end
